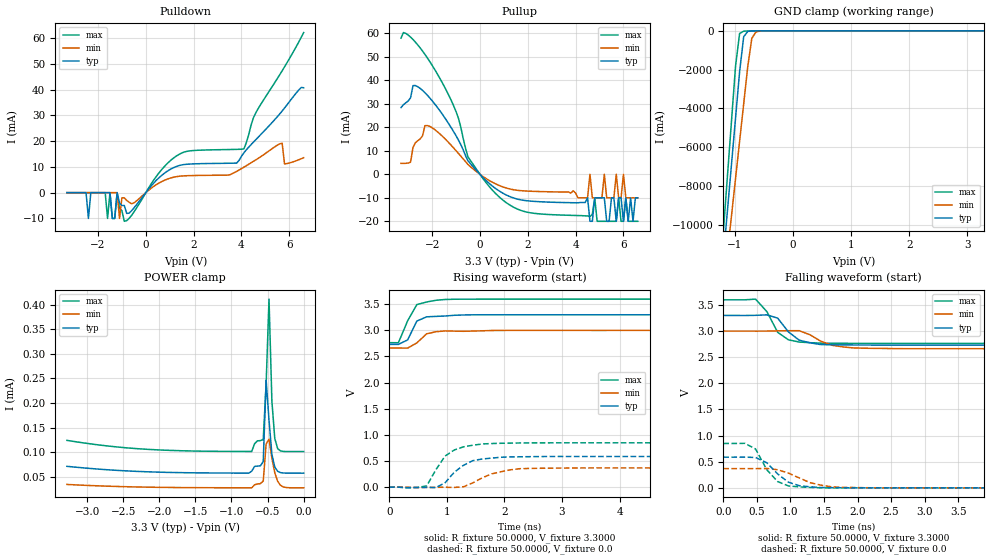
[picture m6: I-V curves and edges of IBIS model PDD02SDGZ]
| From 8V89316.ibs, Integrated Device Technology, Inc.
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|   Model PDD02SDGZ
[Model]  PDD02SDGZ
Model_type I/O
Polarity   Non-Inverting
Enable   Active-Low
Vinl =   0.8000V
Vinh =   2.0000V
Vmeas =  1.6500V
Cref =   50.0000pF
Rref =   1.0000M
Vref =   0.0V
C_comp   2.6301pF   2.6149pF   2.6344pF
[Temperature Range]   25.0000   0.1250k   -40.0000
[Voltage Range]   3.3000V   3.0000V   3.6000V
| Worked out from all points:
|   slope of the pulldown table from 0 to 0.495 V, typ, clamps not added: 93.5 ohm
|   slope of the pullup table from 0 to 0.495 V, typ, clamps not added: 103 ohm
|   GND clamp passes 1 mA (typ) near -0.64 V on its own axis
|   rising waveform, R_fixture 50.0000, V_fixture 3.3000: 20-80 % time 162ps typ, 217ps min, 224ps max; typ from 2.73 V to 3.3 V
|   rising waveform, R_fixture 50.0000, V_fixture 0.0: 20-80 % time 386ps typ, 505ps min, 359ps max; typ from 0 V to 0.587 V
|   falling waveform, R_fixture 50.0000, V_fixture 3.3000: 20-80 % time 263ps typ, 330ps min, 253ps max; typ from 3.3 V to 2.73 V
|   falling waveform, R_fixture 50.0000, V_fixture 0.0: 20-80 % time 304ps typ, 439ps min, 267ps max; typ from 0.587 V to 0 V
[Pulldown]
|Voltage   I(typ)   I(min)   I(max)
-3.3V     0A         0A         0A
-2.5V     0A         0A         0A
-2.4V     -10mA      0A         0A
-1.6V     0A         0A         -10mA
-1.5V     0A         0A         0A
-1.4V     -10mA      0A         -10mA
-1.2V     0A         0A         0A
-1.1V     -4mA       -10mA      -6mA
-900mV    -5mA       -2mA       -11.12mA
1.3V      10.23mA    6.236mA    14.35mA
4.1V      15.46mA    9.887mA    16.97mA
6.6V      40.7mA     13.55mA    62.12mA
[Pullup]
|Voltage   I(typ)   I(min)   I(max)
-3.3V     28.44mA    4.665mA    57.97mA
-2.2V     33.67mA    20.77mA    49.54mA
-500mV    5.727mA    4.156mA    7.397mA
1V        -8.272mA   -5.504mA   -11.3mA
4.5V      -10mA      -10mA      -17.71mA
4.6V      -20mA      0A         -18mA
4.7V      -20mA      -10mA      -17mA
4.8V      -10mA      -10mA      -10mA
6V        -20mA      0A         -20mA
6.1V      -10mA      -10mA      -10mA
6.2V      -20mA      -10mA      -20mA
6.6V      -10mA      -10mA      -20mA
[GND_clamp]
|Voltage   I(typ)   I(min)   I(max)
-3.3V     -83.46A    -71.04A    -95.7A
-1.2V     -11.69A    -13.39A    -10.37A
-1.13V    -9.3A      -11.47A    -7.522A
-1.06V    -6.904A    -9.549A    -4.675A
-990mV    -4.509A    -7.624A    -1.828A
-920mV    -2.113A    -5.699A    -140.8mA
-850mV    -308.3mA   -3.775A    -17.65mA
-780mV    -30.2mA    -1.85A     -8.739mA
-710mV    -4.257mA   -388.3mA   -4.589mA
-640mV    -860.9uA   -62.95mA   -1.764mA
-430mV    -30.34uA   -259.4uA   -43.6uA
3.28V     57.9uA     29.96uA    101.7uA
[POWER_clamp]
|Voltage   I(typ)   I(min)   I(max)
-3.28V    71.8uA     35.04uA    124.4uA
-2.16V    60.67uA    29.52uA    106.2uA
-720mV    61.92uA    28.24uA    101.9uA
-680mV    71.62uA    34.23uA    117.6uA
-560mV    81.4uA     41.98uA    126.2uA
-520mV    246.8uA    117.1uA    238.3uA
-480mV    165.1uA    126.9uA    410.9uA
-440mV    95.81uA    87.83uA    203.3uA
-400mV    70.17uA    58.68uA    128.2uA
-360mV    61.63uA    41.35uA    107.7uA
-320mV    58.98uA    33.21uA    103uA
0V        57.91uA    28.11uA    101.8uA
[Ramp]
| variable   typ   min   max
dV/dt_r  0.3522/0.3861n   0.2209/0.4950n   0.5092/0.3593n
dV/dt_f  0.3402/0.2630n   0.2022/0.3206n   0.4998/0.2504n
R_load = 50.0000
[Rising Waveform]
R_fixture= 50.0000
V_fixture= 3.3000
V_fixture_min= 3.0000
V_fixture_max= 3.6000
L_fixture= 0.0H
C_fixture= 0.0F
|time   V(typ)   V(min)   V(max)
0s        2.731V     2.662V     2.764V
160ps     2.731V     2.662V     2.763V
320ps     2.817V     2.66V      3.182V
480ps     3.178V     2.76V      3.493V
650ps     3.258V     2.934V     3.542V
810ps     3.267V     2.973V     3.575V
970ps     3.274V     2.989V     3.59V
1.29ns    3.294V     2.982V     3.596V
1.62ns    3.298V     2.991V     3.597V
16ns      3.298V     2.999V     3.597V
[Rising Waveform]
R_fixture= 50.0000
V_fixture= 0.0
V_fixture_min= 0.0
V_fixture_max= 0.0
L_fixture= 0.0H
C_fixture= 0.0F
|time   V(typ)   V(min)   V(max)
0s        6.994uV    7.336uV    6.867uV
650ps     -2.869mV   -5.413mV   22.76mV
810ps     -8.775mV   -2.516mV   333.2mV
970ps     84.85mV    -1.495mV   595.6mV
1.13ns    286.7mV    -5.207mV   711.5mV
1.29ns    419.3mV    8.096mV    771.4mV
1.62ns    539.9mV    181.7mV    826.8mV
2.1ns     579.5mV    331.5mV    842.6mV
2.59ns    585mV      361.2mV    847.6mV
16ns      587mV      368.2mV    848.7mV
[Falling Waveform]
R_fixture= 50.0000
V_fixture= 3.3000
V_fixture_min= 3.0000
V_fixture_max= 3.6000
L_fixture= 0.0H
C_fixture= 0.0F
|time   V(typ)   V(min)   V(max)
0s        3.298V     2.999V     3.597V
480ps     3.3V       2.998V     3.61V
650ps     3.309V     2.999V     3.369V
810ps     3.246V     3.003V     2.975V
970ps     2.983V     3.006V     2.832V
1.13ns    2.825V     3.006V     2.789V
1.45ns    2.741V     2.807V     2.768V
1.78ns    2.735V     2.696V     2.765V
2.59ns    2.731V     2.663V     2.764V
16ns      2.731V     2.662V     2.764V
[Falling Waveform]
R_fixture= 50.0000
V_fixture= 0.0
V_fixture_min= 0.0
V_fixture_max= 0.0
L_fixture= 0.0H
C_fixture= 0.0F
|time   V(typ)   V(min)   V(max)
0s        587mV      368.2mV    848.7mV
320ps     587.3mV    368.1mV    851.8mV
480ps     581.4mV    368.3mV    743.9mV
650ps     477.5mV    370.8mV    342.8mV
810ps     265.1mV    345.7mV    120.3mV
970ps     107.9mV    282.5mV    36.11mV
1.29ns    19.54mV    100.3mV    8.842mV
1.62ns    3.629mV    18.75mV    422.5uV
2.26ns    -63.86uV   528.9uV    94.58uV
16ns      -6.418uV   -7.025uV   16.26uV
